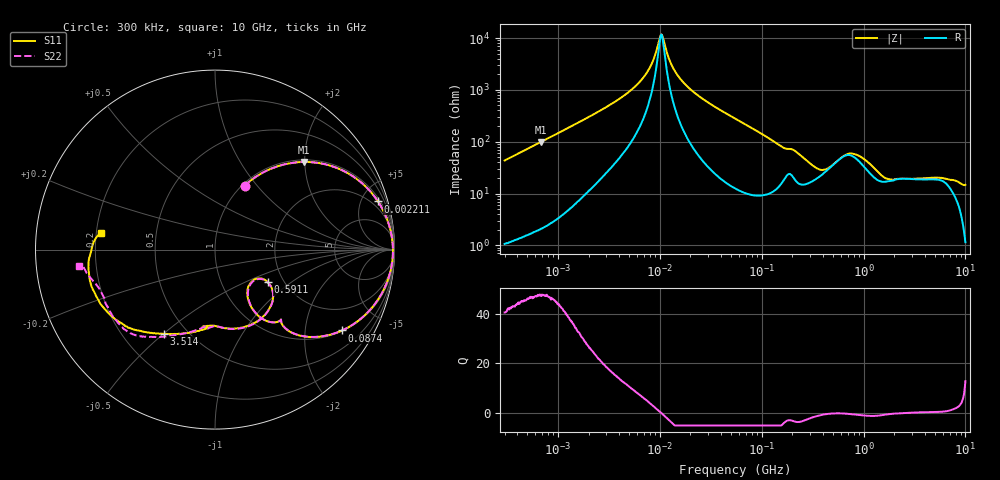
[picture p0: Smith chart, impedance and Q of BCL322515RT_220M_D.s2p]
! S-Parameter Data Generated by TDK Corporation
! Copyright(C) 2024 TDK Corporation.
! All Rights Reserved.
! TDK P/N: BCL322515RT-220M-D (SMD / SMT Inductor (Coil))
! Property: L=22uH at 1MHz
! Size(LxWxT): 3.2x2.5x1.5mm
! Model Type: s2p (Touchstone File Format Version 1.0)
! Frequency: DC=Yes Start=0.3MHz Stop=10000MHz 802points Log-sweep
! Model Generated on May 28, 2024
! Terms and conditions regarding TDK Simulation Models:
! 1)This simulation model is being provided solely for informational
!  purposes. Please refer to the specifications of the products in
!  terms of detailed characteristics of such products.
! 2)In no event shall TDK Corporation of any of its subsidiaries be
!  liable for any loss or damage arising, directly or indirectly,
!  from any information contained in this simulation model, including,
!  but not limited to loss or damages arising from any inaccuracies,
!  omissions or errors in connection with such information.
! 3)Any and all copyrights on this simulation model are owned by
!  TDK Corporation.  Duplication or redistribution of this simulation
!  model without prior written permission from TDK Corporation
!  is prohibited.
! 4)This simulation model is subject to any modification or change
!  without any prior notice.
! 5)Neither TDK Corporation nor any of its subsidiaries shall make any
!  warranty, express or implied, including but not limited to the
!  correctness, implied warranties of merchantability and fitness for
!  a particular purpose with respect to this simulation models.
! 6)The use of this simulation model shall be deemed to have consented
!  to the terms and conditions hereof.
! Port Assignments:
!  1 ---@@@--- 2
! Applicable Conditions:
!  Temperature = 25 degC
!  DC Bias Current = 0 A
!  Small Signal Operation
# Hz S MA R 50
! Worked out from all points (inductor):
!   801 points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, 300 kHz to 10 GHz, reference 50 ohm
!   read as one part in series: L = 23 uH near 318.3 kHz
!   highest Q = 47.5 at 680.6 kHz (marker M1), where L = 23.1 uH
!   self-resonance near 10.27 MHz
!   S11 on the Smith chart (normalised r, x): 300 kHz: 1.03, +0.86; 2.211 MHz: 1.28, +6.68; 87.4 MHz: 1.03, -3.13; 591.1 MHz: 1.66, -0.69; 3.514 GHz: 0.38, -0.50; 10 GHz: 0.22, +0.07
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300000  0.3925 65.2  0.9096 -23.4  0.91 -23.3  0.3927 65.2
680647  0.6949 44.7  0.7044 -44.1  0.7048 -44.1  0.6948 44.7
1713600  0.9199 21.2  0.3631 -66.9  0.3632 -66.9  0.9199 21.2
2211197  0.947 16.4  0.2848 -71.2  0.2851 -71.2  0.947 16.4
6298968  0.9882 3.8  0.07058 -78.5  0.07065 -78.6  0.9882 3.8
8128066  0.9905 1.7  0.03452 -73.5  0.03455 -73.4  0.9907 1.7
9671944  0.9913 0.3  0.01279 -47.7  0.01281 -47.7  0.9914 0.3
1.050326e7  0.9915 -0.4  0.008631 10.9  0.008632 11.0  0.9916 -0.4
1.35567e7  0.9909 -2.5  0.03785 74.8  0.03786 74.8  0.9911 -2.5
1.877128e7  0.9878 -5.5  0.08604 78.9  0.08608 78.9  0.9879 -5.5
5.477226e7  0.9292 -20.9  0.3304 66.6  0.3305 66.6  0.9292 -20.8
8.740098e7  0.8397 -32.4  0.4993 54.5  0.4994 54.5  0.8397 -32.4
1.356511e8  0.6712 -45.5  0.6676 37.9  0.6678 37.9  0.6713 -45.4
3.126428e8  0.3456 -57.0  0.8086 9.4  0.8089 9.4  0.3457 -56.6
4.329008e8  0.2707 -41.3  0.7698 -2.4  0.7701 -2.3  0.2751 -41.1
5.911415e8  0.3467 -31.6  0.6677 -8.7  0.6678 -8.7  0.3494 -32.0
1.001841e9  0.4641 -63.3  0.6733 -3.9  0.6734 -3.9  0.4668 -62.9
1.767019e9  0.4246 -93.8  0.7552 -23.3  0.7554 -23.3  0.4281 -91.3
3.514172e9  0.5475 -121.1  0.6383 -52.1  0.6386 -52.1  0.5496 -118.8
6.576072e9  0.6836 -146.8  0.4864 -81.0  0.4863 -81.1  0.6789 -145.8
8.322921e9  0.7147 -169.4  0.4249 -101.0  0.4253 -101.1  0.6967 -164.8
1e10  0.6416 171.6  0.3368 -112.5  0.3366 -112.7  0.761 -173.2
